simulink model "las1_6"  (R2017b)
settings: Solver=VariableStepDiscrete  StartTime=0.0  StopTime=300  MaxStep=10  RelTol=1e-3  AbsTol=1e-3
undefined symbols (not defined in the file): A, B, C, D, g, h0, T

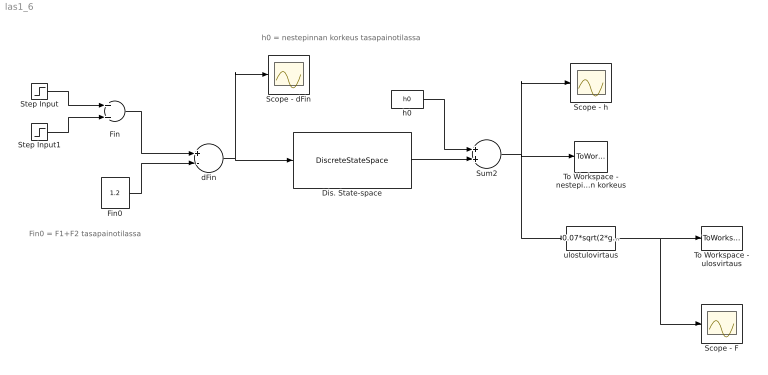
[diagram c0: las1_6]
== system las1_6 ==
  note: Fin0 = F1+F2 tasapainotilassa
  note: h0 = nestepinnan korkeus tasapainotilassa
  Dis. State-space : DiscreteStateSpace  A=A  B=B  C=C  D=D  SampleTime=T
  Fin : Sum
  Fin0 : Constant  Value=1.2
  Scope - F : Scope
  Scope - dFin : Scope
  Scope - h : Scope
  Step Input : Step  Time=10  Before=1.2  After=2.2  SampleTime=0.1
  Step Input1 : Step  Time=15  After=-1  SampleTime=0.1
  Sum2 : Sum
  To Workspace - nestepinnan korkeus : ToWorkspace  VariableName=h
  To Workspace - ulosvirtaus : ToWorkspace  VariableName=F
  dFin : Sum  Inputs=+-
  h0 : Constant  Value=h0
  ulostulovirtaus : Fcn  Expr=0.07*sqrt(2*g*u)
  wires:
  dFin/1 -> Dis. State-space/1, Scope - dFin/1
  Fin0/1 -> dFin/2
  h0/1 -> Sum2/1
  Dis. State-space/1 -> Sum2/2
  Sum2/1 -> To Workspace - nestepinnan korkeus/1, Scope - h/1, ulostulovirtaus/1
  Step Input1/1 -> Fin/2
  Step Input/1 -> Fin/1
  Fin/1 -> dFin/1
  ulostulovirtaus/1 -> To Workspace - ulosvirtaus/1, Scope - F/1
